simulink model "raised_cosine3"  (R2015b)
settings: Solver=VariableStepAuto  StartTime=0.0  StopTime=5  RelTol=1e-3
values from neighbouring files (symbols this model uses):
  hrc = hrc/sum(hrc)    [raised_cosine_1.m]    (also in raised_cosine_2.m = rcosdesign(alpha, n_symb, Tsymb/Ts,'normal'); raised_cosine_3.m = rcosdesign(alpha, n_symb, Tsymb/Ts))
  noise = 0.05    [raised_cosine_3.m]    (also in sgolay_2.m = 0.02; zerophase_1.m = 0.015; zerophase_2.m = 0.01)
  nrc = length(hrc)    [raised_cosine_2.m]    (also in raised_cosine_3.m)
  ns = length(ys(:,1))    [hilbert_filter_1.m]    (also in raised_cosine_1.m = 5; raised_cosine_2.m = 5; raised_cosine_3.m = 5)
  Ts = 1/fs    (= 0.001)    [abtast_fir_1.m]    (also in abtast_fir_2.m; abtast_fir_3.m; abtast_fir_4.m; hilbert_filter_1.m)
  Tsymb = ns*Ts    (= 0.005)    [raised_cosine_1.m]    (also in raised_cosine_2.m; raised_cosine_3.m)
libraries: dspsigops x2, simulink x1

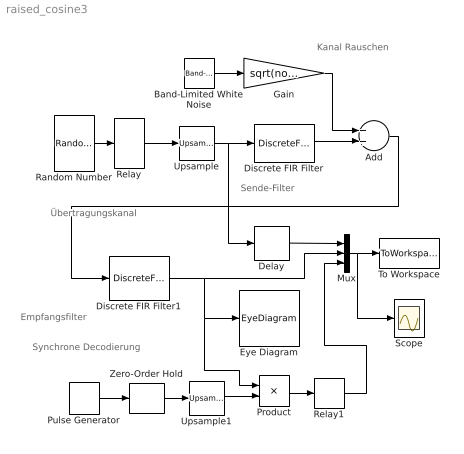
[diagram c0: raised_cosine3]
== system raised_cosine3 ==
  note: Empfangsfilter
  note: Sende-Filter
  note: Synchrone Decodierung
  note: Kanal Rauschen
  note: Übertragungskanal
  Add : Sum
  Band-Limited White Noise : simulink/Sources/Band-Limited White Noise  Cov=Ts  Ts=Ts  seed=[23341]
  Delay : Delay  DelayLength=(nrc-1)
  Discrete FIR Filter : DiscreteFir  Coefficients=hrc  SampleTime=Ts
  Discrete FIR Filter1 : DiscreteFir  Coefficients=hrc  SampleTime=Ts
  Eye Diagram : EyeDiagram
  Gain : Gain  Gain=sqrt(noise)
  Mux : Mux  Inputs=3
  Product : Product
  Pulse Generator : DiscretePulseGenerator  PulseType=Time based  Period=Tsymb  PulseWidth=50
  Random Number : RandomNumber  SampleTime=Tsymb
  Relay : Relay  OffOutputValue=-1
  Relay1 : Relay  OnSwitchValue=0.1  OffSwitchValue=-0.1  OffOutputValue=-1
  Scope : Scope
  To Workspace : ToWorkspace  VariableName=y  SaveFormat=Timeseries  SampleTime=-1
  Upsample : dspsigops/Upsample  N=ns  phase=0  RateOptions=Allow multirate processing  ic=0  mode=Unused parameter value
  Upsample1 : dspsigops/Upsample  N=ns  phase=0  RateOptions=Allow multirate processing  ic=0  mode=Unused parameter value
  Zero-Order Hold : ZeroOrderHold  SampleTime=Tsymb
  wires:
  Random Number/1 -> Relay/1
  Upsample/1 -> Delay/1, Discrete FIR Filter/1
  Relay/1 -> Upsample/1
  Discrete FIR Filter/1 -> Add/2
  Band-Limited White Noise/1 -> Gain/1
  Gain/1 -> Add/1
  Add/1 -> Discrete FIR Filter1/1
  Discrete FIR Filter1/1 -> Eye Diagram/1, Product/1, Mux/2
  Mux/1 -> Scope/1, To Workspace/1
  Delay/1 -> Mux/1
  Pulse Generator/1 -> Zero-Order Hold/1
  Upsample1/1 -> Product/2
  Product/1 -> Relay1/1
  Relay1/1 -> Mux/3
  Zero-Order Hold/1 -> Upsample1/1
